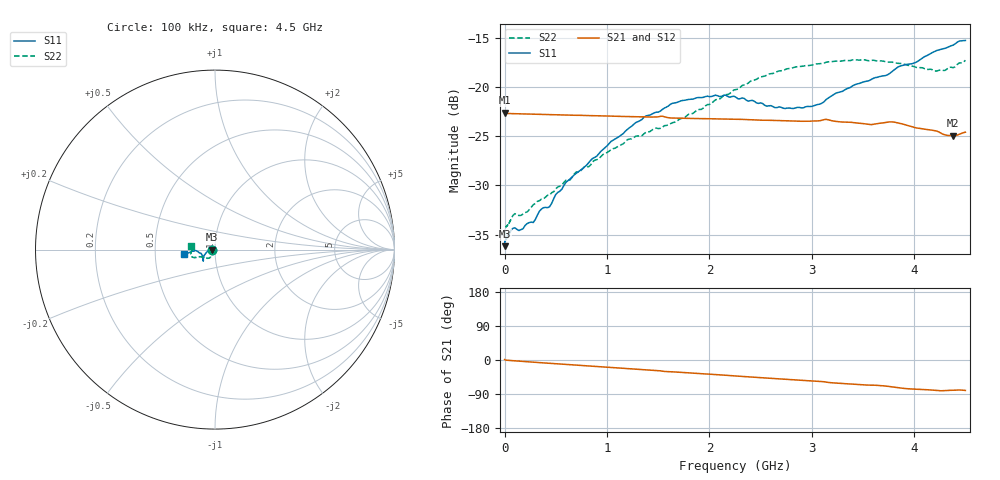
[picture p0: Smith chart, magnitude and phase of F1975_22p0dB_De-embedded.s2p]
! Integrated Device Technology
! Corporate Headquarters
! 6024 Silver Creek Valley Road
! San Jose, CA 95138  USA
! Phone:  1-408-284-8200
! Toll Free:  1-800-223-1366
! Webpage:  http://www.idt.com/
! Timing and RF Division
! 515 Groton Road, Suite 102
! Westford, MA 01886-6024
! Device:  F1975
! Description: 6-bit, 75 ohm, 0.5 dB Digital Step Attenuator
! Frequency:  5.0 MHz -  3.00 GHz
! Package:  4x4 mm QFN Plastic Package: 20 pin
! Ports:  2 RF, 11 DC
!  Pin  1  = D5 (16 dB)
!  Pin  2  = RF1  =  Port 1
!  Pin  3  = Serial Data In (DATA)
!  Pin  4  = Serial Clock (CLK)
!  Pin  5  = Serial Latch Enable (LE)
!  Pin  6  = VDD
!  Pin  7  = NC
!  Pin  8  = NC
!  Pin  9  = NC
!  Pin 10  = GND
!  Pin 11  = GND
!  Pin 12  = NC
!  Pin 13  = VMODE
!  Pin 14  = RF2  =  Port 2
!  Pin 15  = D4 (8 dB)
!  Pin 16  = D3 (4 dB)
!  Pin 17  = D2 (2 dB)
!  Pin 18  = NC
!  Pin 19  = D1 (1 dB)
!  Pin 20  = D0 (0.5 dB)
! State:  44
! Atten State:  22.0 dB
! Voltage:  +3.30 Volts
! Current:  0.591 mA
! Data:  The device was measured on a F1975 evaluation board which has
!  individual transmission lines to the RF pins.  Data was collected
!  using a calibrated network analyzer.  The evaluation board was
!  de-embedded using Automatic Fixture Removal (AFR).
!  The reference plane is the edge of the package pin.
! Misc:
!  Action Tracker AT0415
! Date Measured:  2018-02-08
! Date:  2018-03-26  MJV
! Note:
!  Integrated Device Technology supplies this data as a sample of measured
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# GHz S dB R 75
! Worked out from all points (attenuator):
!   291 points, 100 kHz to 4.5 GHz, reference 75 ohm
!   highest |S21| = -22.61 dB at 100 kHz (marker M1); lowest = -24.9 dB at 4.38 GHz (marker M2)
!   lowest |S11| = -36.2 dB at 100 kHz (marker M3), VSWR 1.03, Z = 72.7 - j0.00957 ohm
!   |S11| at or under -10 dB: start of sweep to end of sweep
!   |S22| runs from -35.1 to -17.2 dB; largest |S21 - S12| = 0.00016
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0.0001  -36.18 -179.8  -22.61 1.2  -22.61 1.2  -35.07 -178.9
0.002  -35.77 -178.6  -22.66 0.9  -22.64 0.9  -34.59 -177.1
0.013  -35.50 -178.0  -22.68 -0.4  -22.68 -0.4  -34.19 -175.2
0.1  -34.31 -175.3  -22.71 -2.2  -22.71 -2.2  -32.88 -161.7
0.16  -34.51 -177.3  -22.73 -3.4  -22.73 -3.4  -33.05 -154.4
0.28  -33.78 -180.0  -22.76 -5.7  -22.76 -5.7  -31.97 -144.8
0.34  -32.63 178.5  -22.78 -6.9  -22.78 -6.9  -31.57 -139.3
0.44  -32.17 -179.5  -22.80 -8.7  -22.80 -8.8  -30.99 -131.2
0.6  -29.68 -175.8  -22.85 -11.8  -22.85 -11.8  -29.47 -126.4
0.76  -28.32 -169.0  -22.88 -14.8  -22.88 -14.8  -28.32 -123.6
1.28  -23.62 -152.7  -23.02 -24.3  -23.02 -24.3  -25.00 -122.8
1.52  -22.46 -145.5  -22.98 -28.6  -22.98 -28.6  -24.20 -129.5
1.64  -21.65 -142.6  -23.15 -31.2  -23.15 -31.2  -23.62 -133.3
1.88  -21.08 -138.6  -23.20 -35.2  -23.20 -35.2  -22.34 -144.3
2.26  -21.05 -137.3  -23.27 -42.2  -23.27 -42.2  -20.25 -155.2
2.64  -22.10 -147.6  -23.39 -49.0  -23.39 -49.0  -18.55 -158.3
3.02  -21.90 -164.2  -23.45 -55.5  -23.45 -55.5  -17.72 -160.7
3.42  -19.76 -175.6  -23.64 -64.3  -23.63 -64.3  -17.21 -166.3
3.76  -18.62 -175.8  -23.54 -70.1  -23.54 -70.1  -17.46 -172.8
4.2  -16.38 -172.7  -24.44 -79.8  -24.43 -79.8  -18.37 175.5
4.38  -15.74 -170.5  -24.94 -79.9  -24.93 -79.9  -18.03 173.2
4.5  -15.26 -171.9  -24.59 -80.4  -24.58 -80.4  -17.28 170.6
